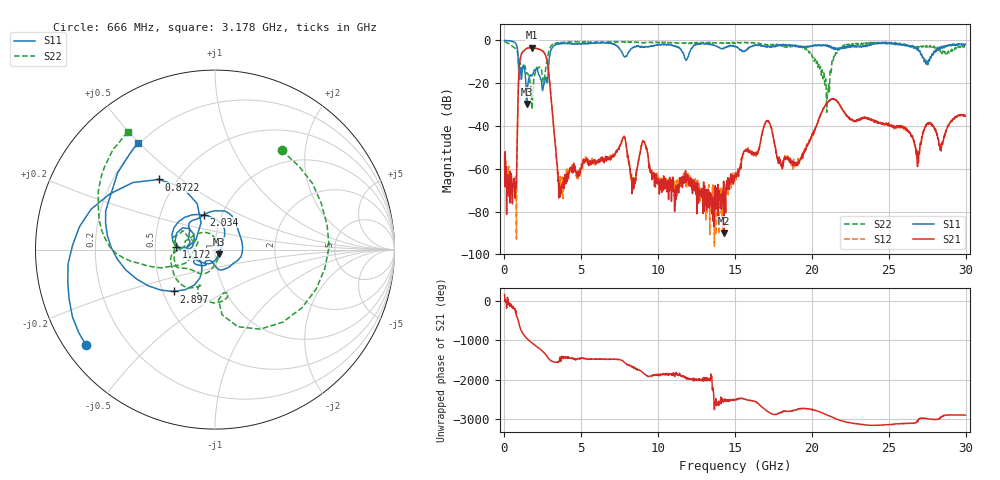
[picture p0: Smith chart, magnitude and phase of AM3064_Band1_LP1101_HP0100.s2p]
# Hz S DB R 50.0
!freq dBS11 angS11 dBS21 angS21 dBS12 angS12 dBS22 angS22
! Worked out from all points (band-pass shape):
!   1600 points, 10 MHz to 29.98 GHz, reference 50 ohm
!   highest |S21| = -3.33 dB at 1.791 GHz (marker M1); lowest = -90.2 dB at 14.27 GHz (marker M2)
!   |S21| within 3 dB of the highest: 1.107 GHz to 2.63 GHz (1.523 GHz wide, 81.5 % of centre)
!   lowest |S11| = -29.7 dB at 1.453 GHz (marker M3), VSWR 1.07, Z = 52.1 - j2.62 ohm
!   |S11| at or under -10 dB: 902.3 MHz to 2.893 GHz (1.99 GHz wide, 105 % of centre); 27.39294 GHz to 27.45987 GHz (66.94 MHz wide, 0.244 % of centre); 27.49127 GHz to 27.56399 GHz (72.72 MHz wide, 0.264 % of centre)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
!   |S22| runs from -33.6 to -0.3 dB; largest |S21 - S12| = 0.01
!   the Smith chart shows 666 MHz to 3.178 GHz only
!   S11 on the Smith chart (normalised r, x): 666 MHz: 0.06, -0.33; 872.2 MHz: 0.40, +0.42; 1.172 GHz: 0.64, +0.02; 2.034 GHz: 0.82, +0.34; 2.897 GHz: 0.57, -0.30; 3.178 GHz: 0.19, +0.50
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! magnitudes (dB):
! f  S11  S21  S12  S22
! 10 MHz  0.0  -53.6  -57.1  -0.3
! 666 MHz  -1.0  -67.1  -65.6  -3.5
! 872.2 MHz  -6.0  -30.9  -30.8  -7.0
! 1.172 GHz  -13.2  -5.5  -5.4  -12.4
! 1.453 GHz  -29.7  -3.7  -3.7  -15.6
! 1.791 GHz  -16.3  -3.3  -3.4  -32.2
! 2.034 GHz  -13.8  -3.7  -3.7  -14.0
! 2.897 GHz  -9.7  -16.0  -15.9  -4.7
! 3.178 GHz  -2.7  -38.6  -38.6  -1.8
! 3.646 GHz  -1.5  -69.8  -69.4  -0.9
! 5.015 GHz  -1.6  -57.7  -59.3  -0.7
! 7.751 GHz  -7.2  -45.1  -45.1  -0.7
! 10 GHz  -2.1  -64.5  -67.5  -1.0
! 14.27 GHz  -3.6  -90.2  -69.1  -1.3
! 15 GHz  -2.9  -63.6  -62.9  -1.4
! 17.07 GHz  -2.9  -37.9  -37.7  -2.1
! 17.97 GHz  -2.4  -58.4  -57.4  -2.2
! 19.99 GHz  -2.8  -44.6  -44.7  -7.0
! 20.98 GHz  -2.3  -29.5  -29.2  -26.3
! 25 GHz  -1.1  -39.6  -39.3  -1.2
! 26.87 GHz  -4.4  -59.0  -54.7  -3.0
! 29.98 GHz  -1.8  -35.4  -35.2  -2.8
